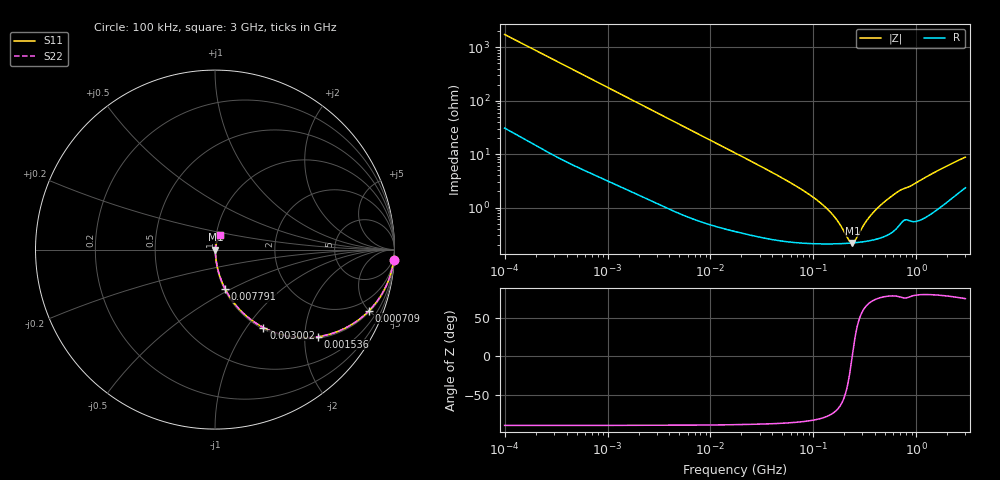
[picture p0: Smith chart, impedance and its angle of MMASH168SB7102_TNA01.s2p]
! MMASH168SB7102_TNA01  S-PARAMETER MODEL  ( Standard Model )
! Model Generated by TAIYO YUDEN Corporation (http://www.ty-top.com)
! Version 1.0
! TAIYO YUDEN Control No. 220601
! Copyright(c) 2013 TAIYO YUDEN CO.,LTD. All Rights Reserved.
! Product Description (link to TY-COMPAS)
! https://ds.yuden.co.jp/TYCOMPAS/or/detail?pn=MMASH168SB7102KTNA01&u=M
! Products Name : Multilayer Ceramic Capacitors
! Characteristics :
!  Capacitance : 1000 [pF] , Rated Voltage : 100 [V] , TCC : X7R
!  Case Size : 1.6 x 0.8 / 0.063 x 0.031 [mm/inch] , Thickness : 0.8 / 0.031 [mm/inch]
!  (Conditions: Temperature = 25 [degC] , DC Bias Voltage = 0 [V])
! External Node Assignments :
!  1  o---| |---o  2
! GND o---------o GND
! Frequency Range : 100kHz  -  3GHz  [ 401 STEP ]
# MHZ S RI R 50
! Freq[MHz].  S11 Real  S11 Imag  S21 Real  S21 Imag  S12 Real  S12 Imag  S22 Real  S22 Imag
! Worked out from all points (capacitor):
!   401 points, 100 kHz to 3 GHz, reference 50 ohm
!   read as one part in series: C = 910 pF near 105.3 kHz
!   lowest |Z| = 218 mohm at 240 MHz (marker M1)
!   series resonance near 238.3 MHz, so ESL is about 490 pH
!   S11 on the Smith chart (normalised r, x): 100 kHz: 2, -35; 709 kHz: 1.09, -5.01; 1.536 MHz: 1.04, -2.33; 3.002 MHz: 1.02, -1.20; 7.791 MHz: 1.01, -0.47; 3 GHz: 1.05, +0.17
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0.1  0.9957 -0.0571  0.00428 0.0571  0.00428 0.0571  0.9957 -0.0571
0.252895  0.9776 -0.14  0.0224 0.14  0.0224 0.14  0.9776 -0.14
0.562235  0.9049 -0.2852  0.0951 0.2852  0.0951 0.2852  0.9049 -0.2852
0.709011  0.8586 -0.34  0.1414 0.34  0.1414 0.34  0.8586 -0.34
1.536162  0.5754 -0.4851  0.4246 0.4851  0.4246 0.4851  0.5754 -0.4851
3.002272  0.27 -0.4341  0.73 0.4341  0.73 0.4341  0.27 -0.4341
3.161081  0.2508 -0.4236  0.7492 0.4236  0.7492 0.4236  0.2508 -0.4236
4.774418  0.1315 -0.3276  0.8685 0.3276  0.8685 0.3276  0.1315 -0.3276
7.79083  0.0566 -0.2195  0.9434 0.2195  0.9434 0.2195  0.0566 -0.2195
17.7727  0.0139 -0.1012  0.9861 0.1012  0.9861 0.1012  0.0139 -0.1012
52.46276  0.00344 -0.0335  0.9966 0.0335  0.9966 0.0335  0.00344 -0.0335
97.38194  0.00236 -0.0159  0.9976 0.0159  0.9976 0.0159  0.00236 -0.0159
150.9232  0.00214 -0.00738  0.9979 0.00738  0.9979 0.00738  0.00214 -0.00738
180.7614  0.00212 -0.00437  0.9979 0.00437  0.9979 0.00437  0.00212 -0.00437
222.1509  0.00215 -0.0011  0.9979 0.0011  0.9979 0.0011  0.00215 -0.0011
240.0085  0.00217 0.000113  0.9978 -0.000113  0.9978 -0.000113  0.00217 0.000113
259.3015  0.0022 0.00132  0.9978 -0.00132  0.9978 -0.00132  0.0022 0.00132
310.5665  0.00231 0.0042  0.9977 -0.0042  0.9977 -0.0042  0.00231 0.0042
362.5028  0.00246 0.00677  0.9975 -0.00677  0.9975 -0.00677  0.00246 0.00677
547.5153  0.00338 0.0147  0.9966 -0.0147  0.9966 -0.0147  0.00338 0.0147
708.4746  0.00545 0.0206  0.9945 -0.0206  0.9945 -0.0206  0.00545 0.0206
3000  0.0296 0.0804  0.9704 -0.0804  0.9704 -0.0804  0.0296 0.0804
